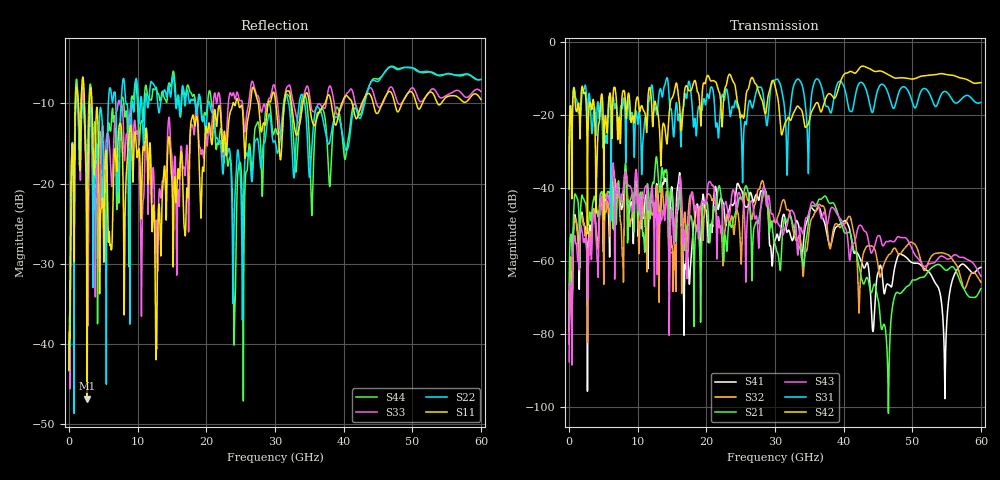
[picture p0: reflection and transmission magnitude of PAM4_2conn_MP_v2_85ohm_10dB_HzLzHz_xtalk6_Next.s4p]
! Info: Touchstone file created by Circ.  Input file=FAB50GbE_2conn_Midplane_Examax_Topo2_v2_85ohm_10dB_HzLzHz.circ
# Hz S RI R 50
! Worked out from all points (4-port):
!   6000 points, 10 MHz to 60 GHz, reference 50 ohm
!   strongest paths, dB at 10 MHz, 15.01 GHz, 30.01 GHz, 45.01 GHz, 60 GHz:
!     S42: -40.1, -15.4, -12.0, -8.0, -11.2
!     S31: -40.3, -20.6, -10.4, -13.0, -16.5
!     S43: -87.6, -46.6, -49.4, -53.1, -64.2
!     S21: -77.6, -41.4, -55.4, -70.4, -67.5
!     S32: -79.2, -55.8, -49.4, -61.0, -65.7
!     S41: -82.7, -40.2, -54.3, -63.2, -61.7
!   lowest |S11| = -46.9 dB at 2.64 GHz (marker M1), VSWR 1.01, Z = 49.7 - j0.334 ohm
!   |S11| at or under -10 dB: 3.332 GHz to 23.87 GHz (20.54 GHz wide, 151 % of centre); 24.68 GHz to 26.42 GHz (1.739 GHz wide, 6.81 % of centre); 35.02 GHz to 37.3 GHz (2.285 GHz wide, 6.32 % of centre)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
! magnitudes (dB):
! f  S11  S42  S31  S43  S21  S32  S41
! 10 MHz  -43.3  -40.1  -40.3  -87.6  -77.6  -79.2  -82.7
! 2.64 GHz  -46.9  -30.9  -22.1  -61.2  -48.8  -62.6  -63.4
! 6.3 GHz  -26.4  -22.2  -16.4  -35.0  -43.3  -38.3  -38.0
! 16.9 GHz  -26.4  -12.6  -14.3  -52.4  -57.1  -47.1  -60.8
! 24.12 GHz  -10.2  -11.5  -16.9  -41.7  -47.7  -50.9  -43.8
! 44.29 GHz  -9.9  -7.9  -19.1  -57.0  -67.1  -56.1  -79.2
! 60 GHz  -9.5  -11.2  -16.5  -64.2  -67.5  -65.7  -61.7
